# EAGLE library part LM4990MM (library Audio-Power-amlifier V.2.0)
LM4990 2 Watt Audio Power Amplifier with Selectable Shutdown Logic Level
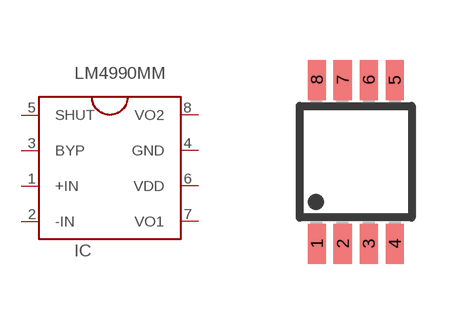
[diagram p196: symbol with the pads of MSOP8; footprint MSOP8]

Designator prefix IC

## LM4990MMLM4990MM_ONLY  [MSOP8]
1  +IN  in
2  -IN  in
3  BYP  in
4  GND  pwr
5  SHUT  in
6  VDD  pwr
7  VO1  out
8  VO2  out

## Footprint MSOP8 (pad centres in mm)
Micro Small Outline Package Grid .65mm
smd 0.45 x 1: 1 -0.975,-2.05; 2 -0.325,-2.05; 3 0.325,-2.05; 4 0.975,-2.05; 5 0.975,2.05; 6 0.325,2.05; 7 -0.325,2.05; 8 -0.975,2.05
